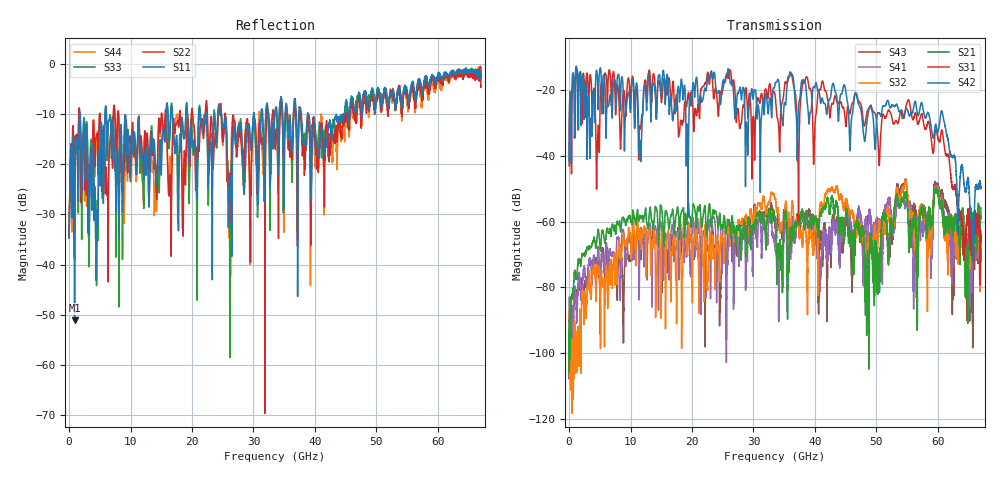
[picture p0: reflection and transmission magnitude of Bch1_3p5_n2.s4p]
!Agilent Technologies,N5247A,US51170199,A.09.90.13
!Agilent N5247A: A.09.90.13
!Date: Wednesday, October 17, 2018 18:16:28
!Correction: S11(Full 4 Port(1,2,3,4))
!S12(Full 4 Port(1,2,3,4))
!S13(Full 4 Port(1,2,3,4))
!S14(Full 4 Port(1,2,3,4))
!S21(Full 4 Port(1,2,3,4))
!S22(Full 4 Port(1,2,3,4))
!S23(Full 4 Port(1,2,3,4))
!S24(Full 4 Port(1,2,3,4))
!S31(Full 4 Port(1,2,3,4))
!S32(Full 4 Port(1,2,3,4))
!S33(Full 4 Port(1,2,3,4))
!S34(Full 4 Port(1,2,3,4))
!S41(Full 4 Port(1,2,3,4))
!S42(Full 4 Port(1,2,3,4))
!S43(Full 4 Port(1,2,3,4))
!S44(Full 4 Port(1,2,3,4))
!S4P File: Measurements: <S11,S12,S13,S14>,
!<S21,S22,S23,S24>,
!<S31,S32,S33,S34>,
!<S41,S42,S43,S44>:
# Hz S  dB  R 50
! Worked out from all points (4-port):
!   6701 points, 10 MHz to 67 GHz, reference 50 ohm
!   strongest paths, dB at 10 MHz, 16.76 GHz, 33.51 GHz, 50.25 GHz, 67 GHz:
!     S42: -41.7, -27.6, -18.3, -27.1, -50.0
!     S31: -43.2, -20.7, -21.5, -35.2, -66.1
!     S21: -89.9, -57.3, -59.2, -72.0, -55.8
!     S32: -87.4, -69.8, -52.8, -64.4, -63.1
!     S41: -83.0, -61.4, -66.0, -60.0, -68.1
!     S43: -89.8, -64.2, -61.2, -63.0, -64.7
!   lowest |S11| = -51.2 dB at 899.9 MHz (marker M1), VSWR 1.01, Z = 49.7 + j0.0966 ohm
!   |S11| at or under -10 dB: 6.075 GHz to 15.81 GHz (9.73 GHz wide, 88.9 % of centre); 24.78 GHz to 30 GHz (5.219 GHz wide, 19.1 % of centre); 37.8 GHz to 43.48 GHz (5.68 GHz wide, 14 % of centre)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
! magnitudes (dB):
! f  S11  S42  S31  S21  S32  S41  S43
! 10 MHz  -34.4  -41.7  -43.2  -89.9  -87.4  -83.0  -89.8
! 899.9 MHz  -51.2  -31.3  -24.7  -75.2  -94.4  -80.0  -81.3
! 4.649 GHz  -31.1  -18.3  -34.1  -63.6  -74.8  -69.7  -71.8
! 6.359 GHz  -12.0  -25.1  -17.1  -63.3  -81.9  -75.5  -70.1
! 26.19 GHz  -24.9  -17.4  -13.9  -62.6  -65.9  -62.1  -62.8
! 55.18 GHz  -6.8  -26.9  -23.1  -60.5  -54.4  -55.9  -58.0
! 67 GHz  -2.8  -50.0  -66.1  -55.8  -63.1  -68.1  -64.7
